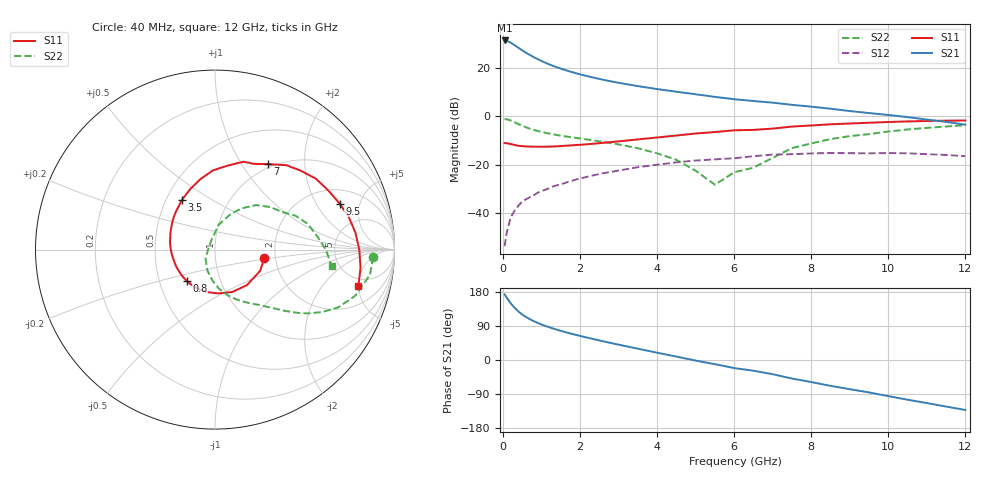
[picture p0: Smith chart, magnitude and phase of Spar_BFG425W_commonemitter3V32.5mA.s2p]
! Filename: 332bfg425.001
! BFG425W Field C1
! V1=8.569E-001V,V2=3.000E+000V, I1=4.679E-004A, I2=3.255E-002A
# GHz  S  MA  R 50
!  S11  S21  S12  S22
!Freq(GHz)  Mag  Ang  Mag  Ang  Mag  Ang  Mag  Ang
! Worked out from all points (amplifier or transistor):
!   44 points, 40 MHz to 12 GHz, reference 50 ohm
!   highest |S21| = 31.6 dB at 40 MHz (marker M1)
!   |S21| within 3 dB of that: start of sweep to 393.2 MHz
!   unconditionally stable (mu >= 1): start of sweep to 71.78 MHz; 978.9 MHz to end of sweep
!   at 700 MHz: K = 0.90, MSG = 29.5 dB, |S12| = -33.6 dB
!   at 2.4 GHz: K = 1.20, MAG = 17.4 dB, |S12| = -24.3 dB
!   at 12 GHz: K = 1.38, MAG = 2.9 dB, |S12| = -16.5 dB
!   S11 on the Smith chart (normalised r, x): 40 MHz: 1.75, -0.18; 800 MHz: 0.69, -0.26; 3.5 GHz: 0.60, +0.38; 7 GHz: 0.95, +1.31; 9.5 GHz: 2.84, +3.22; 12 GHz: 3.98, -4.98
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0.04  0.279 -9.9  38.13 173.0  0.002 67.1  0.881 -2.7
0.1  0.278 -25.2  37.25 163.7  0.004 76.8  0.875 -9.2
0.2  0.266 -48.2  34.19 149.3  0.008 73.3  0.823 -18.1
0.3  0.255 -67.9  30.35 137.7  0.011 70.2  0.758 -25.1
0.4  0.245 -85.3  26.76 128.0  0.014 67.8  0.692 -30.1
0.5  0.241 -100.4  23.67 119.7  0.017 66.0  0.639 -33.8
0.6  0.238 -112.4  21.07 113.0  0.019 64.9  0.593 -36.7
0.8  0.235 -132.0  17.1 102.2  0.023 63.0  0.525 -40.8
1  0.234 -147.1  14.23 93.6  0.028 61.8  0.476 -43.9
1.3  0.237 -164.5  11.29 83.0  0.035 59.7  0.425 -48.3
1.7  0.248 177.4  8.792 71.3  0.044 56.5  0.377 -53.8
2.2  0.265 159.5  6.849 58.7  0.056 51.3  0.33 -61.5
2.8  0.293 141.5  5.378 44.8  0.07 44.0  0.278 -71.4
3.5  0.333 123.6  4.278 29.8  0.088 34.3  0.218 -84.4
4.5  0.401 101.7  3.269 9.0  0.111 19.3  0.125 -109.7
5.5  0.474 81.2  2.555 -11.1  0.128 3.6  0.038 175.3
6.5  0.525 65.4  2.096 -28.3  0.149 -8.9  0.086 92.5
7  0.559 58.4  1.935 -37.5  0.161 -16.7  0.138 82.3
8.5  0.687 35.1  1.448 -68.2  0.174 -45.6  0.338 47.2
9.5  0.74 20.3  1.176 -85.6  0.171 -62.1  0.429 29.2
10.5  0.788 6.9  0.969 -104.8  0.171 -80.4  0.537 15.4
12  0.824 -14.1  0.673 -131.9  0.149 -109.8  0.657 -8.2
